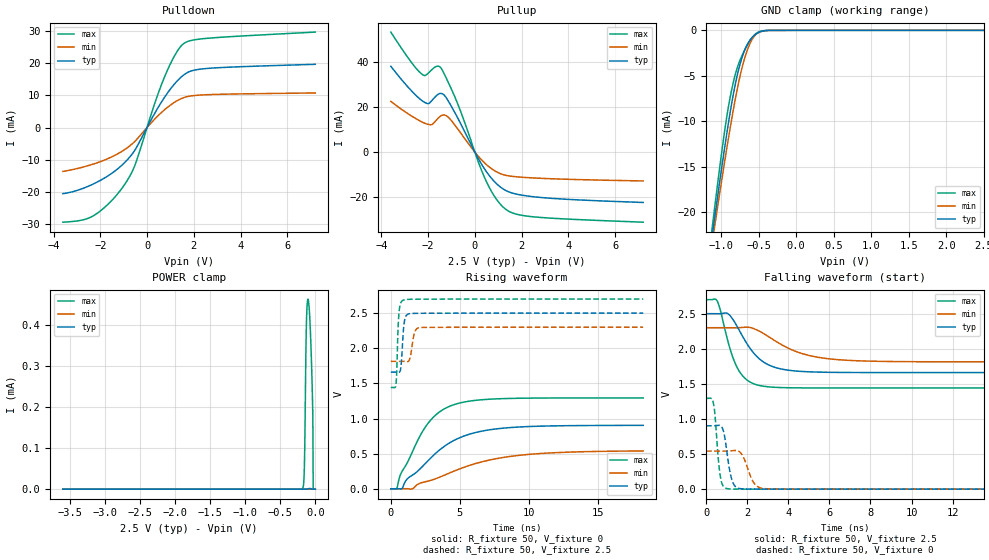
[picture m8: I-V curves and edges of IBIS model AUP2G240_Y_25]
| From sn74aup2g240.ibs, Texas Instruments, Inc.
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[Model]   AUP2G240_Y_25
Model_type  3-state
Enable   Active-Low
Vref =   0
Rref =   1E6
Cref =   30p
Vmeas =   1.25
| variable   typ   min   max
C_comp   2.07pF   1.87pF   2.43pF
| C_pullup   3.00pF   2.04pF   3.80pF
| C_pulldown   2.41pF   2.20pF   2.85pF
| C_tri-state   2.07pF   1.87pF   2.43pF
[Temperature Range]   40   100   -40
| Ambient temperature   25   85   -40
[Voltage range]   2.5   2.3   2.7
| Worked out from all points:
|   slope of the pulldown table from 0 to 0.375 V, typ, clamps not added: 75.2 ohm
|   slope of the pullup table from 0 to 0.375 V, typ, clamps not added: 55.1 ohm
|   GND clamp passes 1 mA (typ) near -0.61 V on its own axis
|   rising waveform, R_fixture 50, V_fixture 0: 20-80 % time 3.49ns typ, 5.05ns min, 2.32ns max; typ from 0 V to 0.902 V
|   falling waveform, R_fixture 50, V_fixture 2.5: 20-80 % time 1.23ns typ, 2.05ns min, 809ps max; typ from 2.5 V to 1.66 V
|   rising waveform, R_fixture 50, V_fixture 2.5: 20-80 % time 175ps typ, 250ps min, 138ps max; typ from 1.66 V to 2.5 V
|   falling waveform, R_fixture 50, V_fixture 0: 20-80 % time 294ps typ, 434ps min, 217ps max; typ from 0.903 V to 0 V
[GND Clamp]
| AUP2G240_Y_25
|   Voltage   I(typ)   I(min)   I(max)
-3.6V     -191.7mA   -177.9mA   -208.5mA
-1.13V    -23.31mA   -24.02mA   -22.49mA
-1.105V   -21.79mA   -22.63mA   -20.79mA
-1.08V    -20.28mA   -21.25mA   -19.11mA
-935mV    -11.93mA   -13.53mA   -10.08mA
-880mV    -9.063mA   -10.78mA   -7.396mA
-820mV    -6.304mA   -7.971mA   -5.14mA
-745mV    -3.66mA    -4.925mA   -3.232mA
-665mV    -1.768mA   -2.52mA    -1.842mA
-585mV    -775.9uA   -970.6uA   -785.9uA
-495mV    -220.6uA   -214.9uA   -155.7uA
2.5V      202.5pA    2.451nA    47.26pA
[POWER Clamp]
| AUP2G240_Y_25
|   Voltage   I(typ)   I(min)   I(max)
-3.6V     1.825nA    3.203nA    718.7pA
-185mV    1.122nA    3.026nA    850.5nA
-165mV    3.482nA    4.861nA    16.25uA
-155mV    8.392nA    6.83nA     59uA
-130mV    101.6nA    18.55nA    377.6uA
-120mV    261.8nA    26.2nA     438.5uA
-105mV    817.7nA    35.95nA    463.9uA
-80mV     1.643uA    34.75nA    421.7uA
-50mV     373.7nA    9.392nA    284.8uA
-35mV     445.8pA    2.866nA    176.4uA
-30mV     389.2pA    1.958nA    59.69pA
0V        0A         0A         0A
[Pulldown]
| AUP2G240_Y_25
|   Voltage   I(typ)   I(min)   I(max)
-3.6V     -20.53mA   -13.63mA   -29.37mA
-2.775V   -18.98mA   -12.34mA   -28.71mA
-2.265V   -17.4mA    -11.26mA   -27.25mA
-1.575V   -14.54mA   -9.325mA   -23.13mA
-965mV    -10.92mA   -6.876mA   -17.74mA
-505mV    -6.845mA   -4.178mA   -11.45mA
310mV     4.162mA    2.467mA    7.071mA
775mV     9.655mA    5.67mA     16.13mA
1.215V    13.84mA    8.012mA    22.73mA
1.565V    16.29mA    9.252mA    26.03mA
2.59V     18.34mA    10.19mA    27.69mA
7.2V      19.61mA    10.73mA    29.61mA
[Pullup]
| AUP2G240_Y_25
|   Voltage   I(typ)   I(min)   I(max)
-3.6V     38.06mA    22.49mA    53.18mA
-2.25V    22.71mA    13.32mA    34.41mA
-1.85V    22.81mA    12.24mA    36.49mA
-1.605V   25.46mA    14.72mA    38.11mA
-1.43V    25.99mA    16.26mA    36.93mA
-1.09V    21.76mA    14.99mA    29.76mA
-655mV    13.52mA    9.171mA    19.24mA
455mV     -8.051mA   -5.133mA   -12.19mA
885mV     -13.53mA   -8.435mA   -20.28mA
1.32V     -16.93mA   -10.21mA   -25.25mA
2.555V    -19.74mA   -11.4mA    -28.63mA
7.2V      -22.22mA   -12.7mA    -30.95mA
[Ramp]
| AUP2G240_Y_25
| variable   typ   min   max
dV/dt_r   0.54/3.49E-09   0.33/5.10E-09   0.78/2.32E-09
dV/dt_f   0.51/1.23E-09   0.30/2.06E-09   0.76/8.13E-10
R_load = 50
[Rising Waveform]
| AUP2G240_Y_25
R_fixture =   50
C_fixture =   0
L_fixture =   0
V_fixture =   0
V_fixture_min = 0
V_fixture_max = 0
|   Time   V(typ)   V(min)   V(max)
0s        8.96nV     28.07nV    865.3pV
429ps     76.64uV    -10.4uV    6.072mV
745ps     -1.285mV   -11.43uV   221.7mV
1.193ns   140.4mV    816.6uV    370.9mV
2.637ns   387.7mV    106.5mV    915.8mV
3.445ns   538.4mV    158mV      1.082V
4.425ns   671.9mV    238.8mV    1.187V
6.537ns   818.3mV    380.6mV    1.266V
9.389ns   880.2mV    477.7mV    1.288V
18.29ns   902.5mV    538.5mV    1.293V
[Falling Waveform]
| AUP2G240_Y_25
R_fixture =   50
C_fixture =   0
L_fixture =   0
V_fixture =   2.5
V_fixture_min = 2.3
V_fixture_max = 2.7
|   Time   V(typ)   V(min)   V(max)
0s        2.5V       2.3V       2.7V
557ps     2.499V     2.3V       2.67V
1.101ns   2.491V     2.3V       2.064V
1.389ns   2.379V     2.299V     1.811V
1.713ns   2.211V     2.303V     1.638V
2.609ns   1.852V     2.248V     1.476V
3.321ns   1.738V     2.12V      1.452V
4.373ns   1.683V     1.962V     1.443V
6.193ns   1.664V     1.85V      1.442V
18.29ns   1.661V     1.814V     1.442V
[Rising Waveform]
| AUP2G240_Y_25
R_fixture =   50
C_fixture =   0
L_fixture =   0
V_fixture =   2.5
V_fixture_min = 2.3
V_fixture_max = 2.7
|   Time   V(typ)   V(min)   V(max)
0s        1.661V     1.814V     1.442V
361ps     1.661V     1.814V     1.462V
421ps     1.661V     1.814V     1.631V
553ps     1.659V     1.814V     2.395V
689ps     1.679V     1.814V     2.628V
941ps     2.315V     1.814V     2.687V
1.333ns   2.491V     1.829V     2.696V
1.721ns   2.496V     2.221V     2.698V
2.077ns   2.497V     2.293V     2.698V
18.29ns   2.5V       2.3V       2.7V
[Falling Waveform]
| AUP2G240_Y_25
R_fixture =   50
C_fixture =   0
L_fixture =   0
V_fixture =   0
V_fixture_min = 0
V_fixture_max = 0
|   Time   V(typ)   V(min)   V(max)
0s        902.9mV    542.1mV    1.293V
349ps     902.9mV    542mV      1.232V
693ps     906.9mV    541.6mV    180.8mV
853ps     817.1mV    541.8mV    36.85mV
1.005ns   544.1mV    542.7mV    8.957mV
1.281ns   111.8mV    548mV      1.633mV
1.677ns   6.767mV    520.1mV    564.4uV
2.301ns   1.081mV    101.2mV    174.8uV
2.801ns   474.5uV    8.795mV    74.36uV
18.29ns   36.31nV    89.02nV    5.672nV
